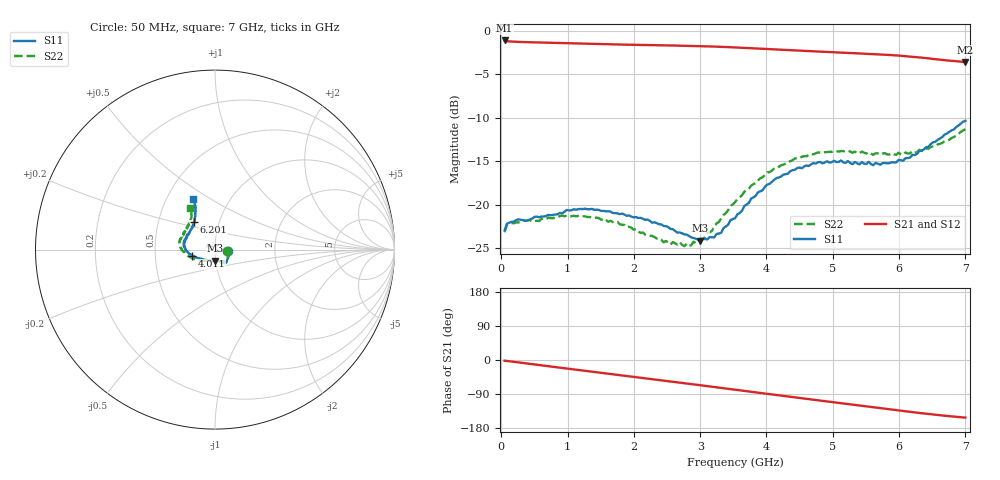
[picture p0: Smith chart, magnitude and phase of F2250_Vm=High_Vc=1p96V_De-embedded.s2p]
! Integrated Device Technology
! Corporate Headquarters
! 6024 Silver Creek Valley Road
! San Jose, CA 95138  USA
! Phone:  1-408-284-8200
! Toll Free:  1-800-223-1366
! Webpage:  http://www.idt.com/
! Timing and RF Division
! 515 Groton Road, Suite 102
! Westford, MA 01886-6024
! Device:  F2250
! Description: Voltage Variable RF Attenuator
! Frequency:  50.0 -  6000.00 MHz
! Package:  3x3 mm Thin QFN Plastic Package: 16 pin
! Ports:  2 RF, 3 DC
!  Pin  1  = GND
!  Pin  2  = NC
!  Pin  3  = RF1  = Port 1
!  Pin  4  = NC
!  Pin  5  = GND
!  Pin  6  = GND
!  Pin  7  = GND
!  Pin  8  = GND
!  Pin  9  = NC
!  Pin 10  = RF2  = Port 2
!  Pin 11  = NC
!  Pin 12  = GND
!  Pin 13  = GND
!  Pin 14  = VCNTRL
!  Pin 15  = VDD
!  Pin 16  = VMODE
! Vcntrl:  1.960 Volts
! Vmode:  +3.300 Volts
! Vdd:  +3.30  Volts
! Current:  1.321 mA
! Data:  The device was measured on a the F2250 evaluation board which has
!  individual transmission lines to the RF pins.  Data was collected
!  using a calibrated network analyzer.  The evaluation board was
!  de-embedded using a TRL calibration technique.
!  The reference plane is the edge of the package pin.
! Misc:  SN 10
!  Action Tracker AT0258
! Date Measured:  2014-11-26
! Date:  2015-10-15  MJV
! Note:
!  Integrated Device Technology supplies this data as a sample of measured
!  data at the package pin for this product.  Your particular data for this
!  product may vary.
!  Data was taken at 25 degrees C.
!  Integrated Device Technology reserves the right to change this data at anytime.
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# GHz S dB R 50
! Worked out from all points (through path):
!   201 points, 50 MHz to 7 GHz, reference 50 ohm
!   highest |S21| = -1.07 dB at 50 MHz (marker M1); lowest = -3.6 dB at 7 GHz (marker M2)
!   group delay of S21, straight-line fit = 61.1 ps
!   lowest |S11| = -24.2 dB at 3.004 GHz (marker M3), VSWR 1.13, Z = 49.7 - j6.18 ohm
!   |S11| at or under -10 dB: start of sweep to end of sweep
!   |S22| runs from -24.8 to -11.3 dB; largest |S21 - S12| = 0.0018
!   S11 on the Smith chart (normalised r, x): 50 MHz: 1.15, -0.02; 4.011 GHz: 0.78, -0.05; 6.201 GHz: 0.76, +0.24; 7 GHz: 0.68, +0.42
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0.05  -22.98 -8.0  -1.07 -1.8  -1.07 -1.8  -23.20 -8.8
0.08475  -22.21 -7.4  -1.15 -2.5  -1.15 -2.5  -22.35 -7.9
0.1195  -22.10 -8.0  -1.19 -3.3  -1.18 -3.3  -22.17 -7.6
0.6755  -21.31 -31.4  -1.33 -15.7  -1.33 -15.7  -21.67 -33.4
1.2315  -20.53 -49.8  -1.45 -27.9  -1.45 -27.9  -21.35 -56.4
1.75275  -21.02 -56.7  -1.54 -39.1  -1.54 -39.1  -22.01 -64.9
2.37825  -22.27 -57.9  -1.63 -52.7  -1.63 -52.7  -23.88 -70.3
2.552  -22.81 -62.0  -1.65 -56.6  -1.65 -56.6  -24.62 -76.8
2.691  -23.23 -68.1  -1.68 -59.7  -1.68 -59.7  -24.33 -83.5
2.7605  -23.44 -69.9  -1.69 -61.2  -1.69 -61.2  -24.80 -87.5
3.00375  -24.16 -89.4  -1.73 -66.7  -1.73 -66.7  -23.95 -107.9
3.21225  -23.78 -110.1  -1.78 -71.4  -1.78 -71.4  -22.48 -125.4
3.525  -21.59 -138.9  -1.87 -78.5  -1.87 -78.5  -19.74 -144.3
3.76825  -19.31 -154.5  -1.97 -84.0  -1.97 -84.0  -17.82 -155.9
4.0115  -17.70 -164.7  -2.06 -89.4  -2.06 -89.4  -16.29 -165.8
4.4285  -15.99 -177.4  -2.22 -98.6  -2.23 -98.6  -14.68 -178.8
4.7065  -15.22 175.0  -2.32 -104.8  -2.33 -104.8  -14.20 175.1
5.054  -15.09 166.7  -2.45 -112.4  -2.45 -112.5  -13.83 167.7
5.85325  -15.22 140.1  -2.75 -129.9  -2.75 -130.0  -14.23 148.5
6.20075  -14.27 127.6  -2.95 -137.6  -2.96 -137.7  -13.86 139.2
6.54825  -12.75 118.8  -3.23 -144.6  -3.23 -144.8  -13.25 127.8
7  -10.34 113.3  -3.55 -152.0  -3.56 -152.1  -11.32 121.3
